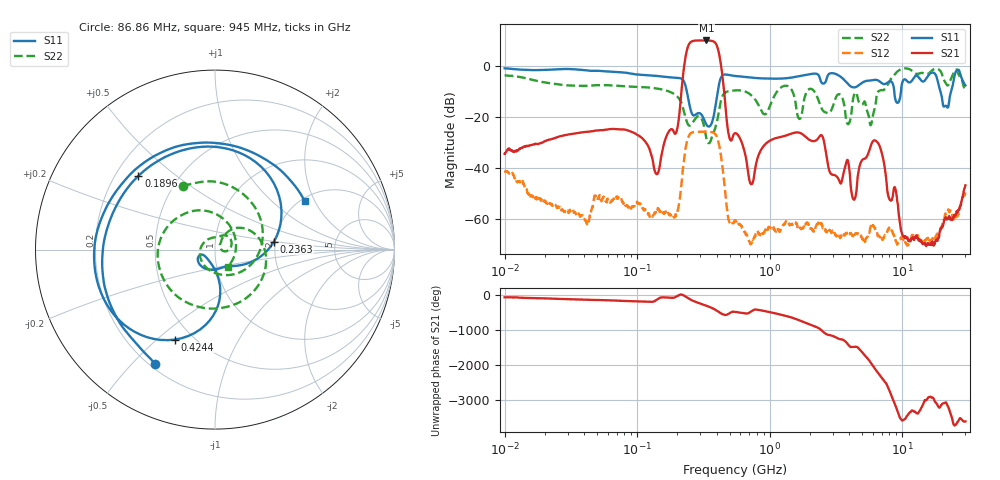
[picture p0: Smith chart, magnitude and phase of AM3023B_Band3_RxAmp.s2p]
# Hz S DB R 50.0
!freq dBS11 angS11 dBS21 angS21 dBS12 angS12 dBS22 angS22
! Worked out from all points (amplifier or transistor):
!   1601 points, 10 MHz to 30 GHz, reference 50 ohm
!   highest |S21| = 10.0 dB at 333.7 MHz (marker M1)
!   |S21| within 3 dB of that: 239.8 MHz to 405.4 MHz (165.6 MHz wide, 51.3 % of centre)
!   unconditionally stable (mu >= 1): start of sweep to end of sweep
!   at 37.85 MHz: K = 2054.19, MAG = -20.0 dB, |S12| = -58.4 dB
!   at 547.7 MHz: K = 5814.94, MAG = -23.6 dB, |S12| = -60.5 dB
!   at 30 GHz: K = 22584.07, MAG = -45.3 dB, |S12| = -49.1 dB
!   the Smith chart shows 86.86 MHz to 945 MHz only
!   S11 on the Smith chart (normalised r, x): 86.86 MHz: 0.22, -0.59; 189.6 MHz: 0.29, +0.37; 236.3 MHz: 1.96, +0.20; 424.4 MHz: 0.40, -0.57; 945 MHz: 2.09, +1.67
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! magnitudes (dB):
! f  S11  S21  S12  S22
! 10 MHz  -0.9  -34.4  -41.0  -3.7
! 38.04 MHz  -1.5  -26.0  -58.7  -7.8
! 86.86 MHz  -2.9  -25.4  -55.5  -8.0
! 144.7 MHz  -4.0  -41.5  -55.9  -8.9
! 189.6 MHz  -4.5  -26.0  -59.3  -10.9
! 236.3 MHz  -9.6  5.7  -30.1  -21.6
! 333.7 MHz  -23.0  10.0  -25.7  -28.5
! 424.4 MHz  -5.2  2.1  -33.5  -14.7
! 490.6 MHz  -3.5  -26.8  -60.2  -9.9
! 547.7 MHz  -3.9  -26.3  -60.5  -9.6
! 724.9 MHz  -4.6  -46.3  -69.5  -11.4
! 945 MHz  -4.9  -30.2  -63.6  -18.5
! 2.084 GHz  -3.1  -29.3  -63.7  -9.1
! 3.914 GHz  -7.1  -37.4  -65.3  -22.8
! 4.326 GHz  -8.4  -52.3  -66.1  -11.5
! 6.36 GHz  -5.4  -29.4  -63.6  -13.3
! 7.926 GHz  -6.2  -51.5  -63.7  -6.7
! 10.38 GHz  -5.2  -67.0  -68.1  -0.9
! 16.96 GHz  -2.6  -68.7  -67.7  -1.6
! 21.24 GHz  -15.6  -59.1  -57.7  -6.6
! 25.82 GHz  -1.7  -56.7  -58.5  -1.5
! 30 GHz  -7.6  -46.7  -49.1  -9.2
